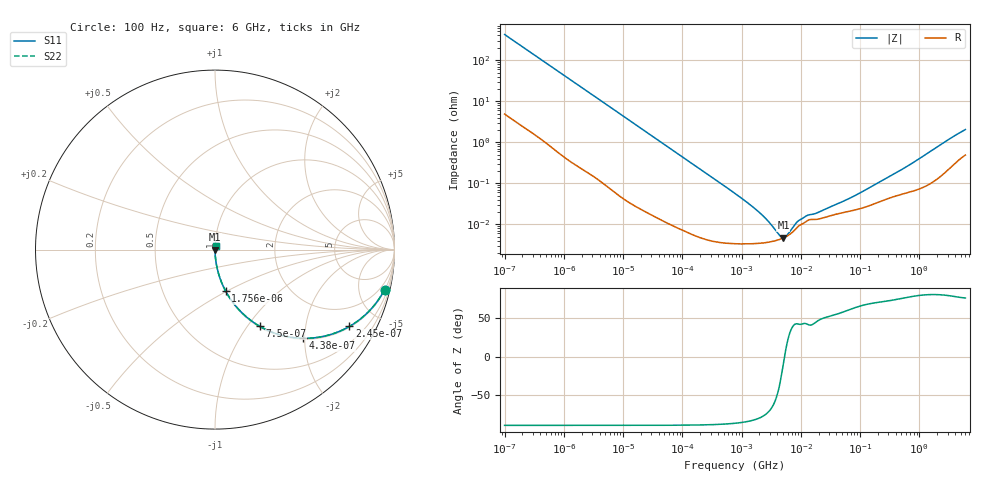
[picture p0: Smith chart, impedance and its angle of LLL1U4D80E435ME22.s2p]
!Murata Part Number: LLL1U4D80E435ME22
!These Parameters are Measured in Series Mode Connection
!Data Generated on Jan 08, 2026
!  o--ll--o
!Port1  Port2
!  o------o
!Operation Temp=25[degC], DC Bias Voltage=0[V]
!Freq. Start=100[Hz] Stop=6[GHz] 401[Steps]
# Hz S RI R 50
!Freq.(Hz) S11(Real) S11(Imag) S21(Real) S21(Imag) S12(Real) S12(Imag) S22(Real) S22(Imag)
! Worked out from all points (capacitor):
!   401 points, 100 Hz to 6 GHz, reference 50 ohm
!   read as one part in series: C = 3.75 uF near 109 Hz
!   lowest |Z| = 4.72 mohm at 5.079 MHz (marker M1)
!   S11 on the Smith chart (normalised r, x): 100 Hz: 1.10, -8.46; 245 Hz: 1.04, -3.48; 438 Hz: 1.02, -1.95; 750 Hz: 1.01, -1.15; 1.756 kHz: 1.01, -0.49; 6 GHz: 1.01, +0.04
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100  0.9448 -0.2227  0.0552 0.2227  0.0552 0.2227  0.9448 -0.2227
164  0.868 -0.3329  0.132 0.3329  0.132 0.3329  0.868 -0.3329
245  0.7493 -0.4277  0.2507 0.4277  0.2507 0.4277  0.7493 -0.4277
438  0.4884 -0.4942  0.5116 0.4942  0.5116 0.4942  0.4884 -0.4942
750  0.2495 -0.4275  0.7505 0.4275  0.7505 0.4275  0.2495 -0.4275
1122  0.1309 -0.3323  0.8691 0.3323  0.8691 0.3323  0.1309 -0.3323
1756  0.0591 -0.2308  0.9409 0.2308  0.9409 0.2308  0.0591 -0.2308
2008  0.0462 -0.2048  0.9538 0.2048  0.9538 0.2048  0.0462 -0.2048
6728  0.00482 -0.0644  0.9952 0.0644  0.9952 0.0644  0.00482 -0.0644
40335  0.000254 -0.0109  0.9997 0.0109  0.9997 0.0109  0.000254 -0.0109
774597  3.39e-05 -0.000564  1 0.000564  1 0.000564  3.39e-05 -0.000564
1734173  3.4e-05 -0.000229  1 0.000229  1 0.000229  3.4e-05 -0.000229
3103719  3.75e-05 -9.42e-05  1 9.42e-05  1 9.42e-05  3.75e-05 -9.42e-05
5079039  4.66e-05 -7.5e-06  1 7.5e-06  1 7.5e-06  4.66e-05 -7.5e-06
7599586  6.86e-05 5.92e-05  0.9999 -5.92e-05  0.9999 -5.92e-05  6.86e-05 5.92e-05
1.243624e7  0.000118 0.000109  0.9999 -0.000109  0.9999 -0.000109  0.000118 0.000109
1.555665e7  0.000131 0.000116  0.9999 -0.000116  0.9999 -0.000116  0.000131 0.000116
6.817316e7  0.00021 0.000384  0.9998 -0.000384  0.9998 -0.000384  0.00021 0.000384
3.124326e8  0.000436 0.00139  0.9996 -0.00139  0.9996 -0.00139  0.000436 0.00139
7.650043e8  0.000646 0.00304  0.9994 -0.00304  0.9994 -0.00304  0.000646 0.00304
3.666503e9  0.00287 0.0131  0.9971 -0.0131  0.9971 -0.0131  0.00287 0.0131
6e9  0.00523 0.0196  0.9948 -0.0196  0.9948 -0.0196  0.00523 0.0196
